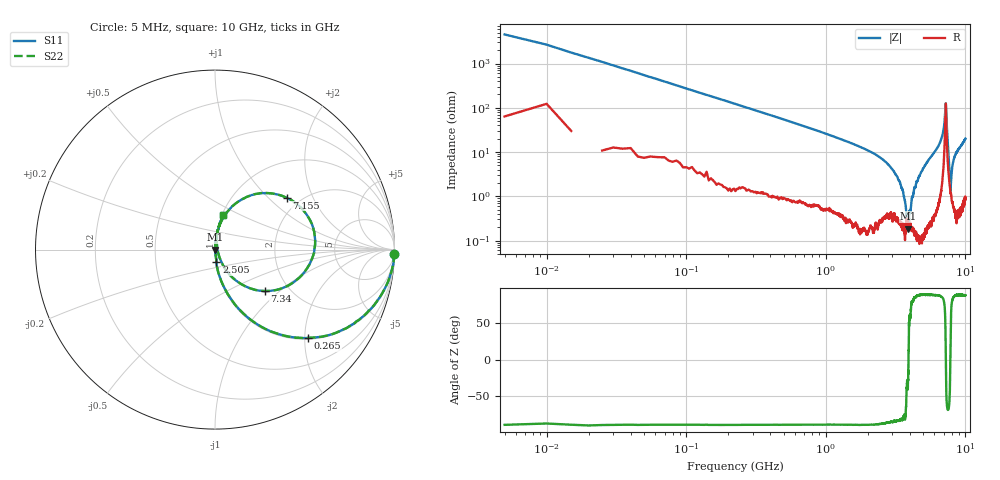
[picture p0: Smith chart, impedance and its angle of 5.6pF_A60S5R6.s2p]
! Amotech Co.,Ltd.
! http://www.amotech.co.kr/
! Part Number: A60S5R6
! These Parameters are Measured in Series Mode Connection
! Operation Temp=25[degC], DC Bias Voltage=0[V]
! Freq. Start=5[MHz] Stop=10[GHz], 2000[Steps]
! Date: Monday, July 13, 2020, 01:30:01
# GHZ S RI R 50.000000
!Freq.(Hz) S11(Real) S11(Imag) S21(Real) S21(Imag) S12(Real) S12(Imag) S22(Real) S22(Imag)
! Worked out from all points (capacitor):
!   2000 points, 5 MHz to 10 GHz, reference 50 ohm
!   read as one part in series: C = 5.83 pF near 55 MHz
!   lowest |Z| = 187 mohm at 3.91 GHz (marker M1)
!   series resonance near 3.915 GHz, so ESL is about 280 pH
!   S11 on the Smith chart (normalised r, x): 5 MHz: 2, -91; 265 MHz: 1.03, -2.07; 2.505 GHz: 1.01, -0.14; 7.155 GHz: 1.70, +1.30; 7.34 GHz: 1.51, -0.80; 10 GHz: 1.02, +0.40
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0.005  0.9992 -0.022  0.000797 0.022  0.000797 0.022  0.9992 -0.022
0.095  0.8879 -0.3077  0.1121 0.3077  0.1121 0.3077  0.8879 -0.3077
0.265  0.5174 -0.4925  0.4826 0.4925  0.4826 0.4925  0.5174 -0.4925
0.69  0.1365 -0.3343  0.8635 0.3343  0.8635 0.3343  0.1365 -0.3343
1.675  0.0214 -0.1369  0.9786 0.1369  0.9786 0.1369  0.0214 -0.1369
2.505  0.00786 -0.0706  0.9921 0.0706  0.9921 0.0706  0.00786 -0.0706
3.34  0.00329 -0.0221  0.9967 0.0221  0.9967 0.0221  0.00329 -0.0221
3.585  0.00182 -0.0122  0.9982 0.0122  0.9982 0.0122  0.00182 -0.0122
3.91  0.00187 -0.000113  0.9981 0.000113  0.9981 0.000113  0.00187 -0.000113
4.14  0.0018 0.00888  0.9982 -0.00888  0.9982 -0.00888  0.0018 0.00888
4.31  0.00154 0.0153  0.9985 -0.0153  0.9985 -0.0153  0.00154 0.0153
5.005  0.00305 0.0434  0.997 -0.0434  0.997 -0.0434  0.00305 0.0434
6.67  0.0427 0.1719  0.9573 -0.1719  0.9573 -0.1719  0.0427 0.1719
6.99  0.1348 0.2706  0.8652 -0.2706  0.8652 -0.2706  0.1348 0.2706
7.155  0.3987 0.2894  0.6013 -0.2894  0.6013 -0.2894  0.3987 0.2894
7.24  0.5545 0.00561  0.4455 -0.00561  0.4455 -0.00561  0.5545 0.00561
7.34  0.2762 -0.231  0.7238 0.231  0.7238 0.231  0.2762 -0.231
7.485  0.0713 -0.1278  0.9287 0.1278  0.9287 0.1278  0.0713 -0.1278
7.805  0.0124 0.00132  0.9876 -0.00132  0.9876 -0.00132  0.0124 0.00132
8.06  0.00969 0.046  0.9903 -0.046  0.9903 -0.046  0.00969 0.046
8.335  0.0099 0.0737  0.9901 -0.0737  0.9901 -0.0737  0.0099 0.0737
10  0.0472 0.1909  0.9528 -0.1909  0.9528 -0.1909  0.0472 0.1909
